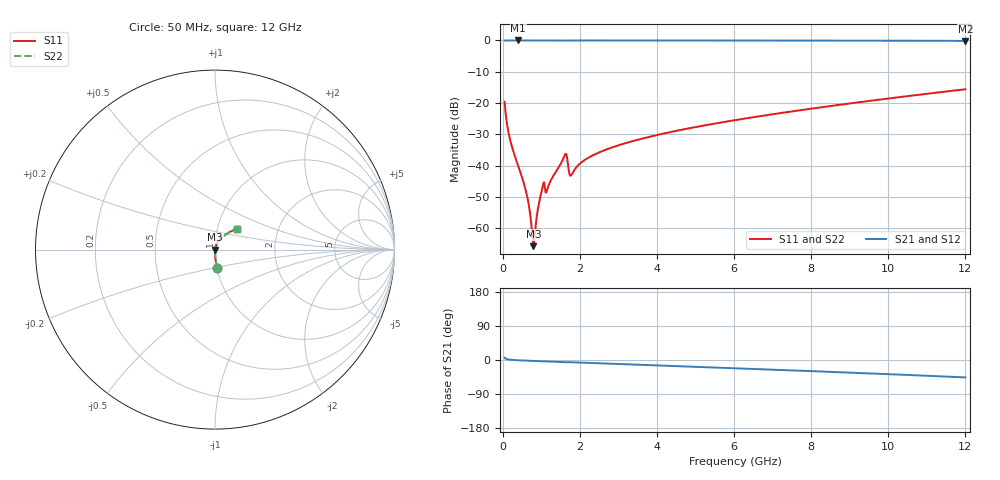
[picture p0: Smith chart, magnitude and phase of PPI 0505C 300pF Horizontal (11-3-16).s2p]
# MHz S MA R 50
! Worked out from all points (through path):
!   1601 points, 50 MHz to 12 GHz, reference 50 ohm
!   highest |S21| = 0.00 dB at 401 MHz (marker M1); lowest = -0.1 dB at 12 GHz (marker M2)
!   group delay of S21, straight-line fit = 10.7 ps
!   lowest |S11| = -65.7 dB at 796.9 MHz (marker M3), VSWR 1.00, Z = 50.1 - j0.00941 ohm
!   |S11| at or under -10 dB: start of sweep to end of sweep
!   |S22| runs from -65.7 to -15.6 dB; largest |S21 - S12| = 0
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50  0.105 -84.0  0.9943 5.9  0.9943 5.9  0.105 -84.0
191.9062  0.02606 -88.5  0.9993 0.9  0.9993 0.9  0.02606 -88.5
401.0312  0.01001 -88.5  0.9995 -0.7  0.9995 -0.7  0.01001 -88.5
625.0938  0.003442 -84.1  0.9995 -1.8  0.9995 -1.8  0.003442 -84.1
684.8438  0.002212 -79.6  0.9995 -2.0  0.9995 -2.0  0.002212 -79.6
759.5312  0.000893 -58.3  0.9995 -2.3  0.9995 -2.3  0.000893 -58.3
796.875  0.0005189 -10.4  0.9994 -2.5  0.9994 -2.5  0.0005189 -10.4
834.2188  0.0007852 44.8  0.9994 -2.7  0.9994 -2.7  0.0007852 44.8
931.3125  0.002338 71.9  0.9993 -3.1  0.9993 -3.1  0.002338 71.9
1035.875  0.004617 70.9  0.9987 -3.5  0.9987 -3.5  0.004617 70.9
1162.844  0.004308 72.4  0.9989 -3.9  0.9989 -3.9  0.004308 72.4
1603.5  0.01447 64.4  0.9949 -5.8  0.9949 -5.8  0.01447 64.4
1648.312  0.01526 45.8  0.9903 -5.9  0.9903 -5.9  0.01526 45.8
1737.938  0.00715 42.7  0.9951 -5.8  0.9951 -5.8  0.00715 42.7
1775.281  0.00704 58.0  0.9968 -5.9  0.9968 -5.9  0.00704 58.0
2044.156  0.01132 77.5  0.9987 -7.1  0.9987 -7.1  0.01132 77.5
2768.625  0.01889 77.5  0.9987 -9.7  0.9987 -9.7  0.01889 77.5
4038.312  0.03123 73.8  0.9983 -14.4  0.9983 -14.4  0.03123 73.8
6025  0.05336 67.0  0.997 -21.8  0.997 -21.8  0.05336 67.0
8019.156  0.08167 59.6  0.9948 -29.4  0.9948 -29.4  0.08167 59.6
10013.31  0.1185 51.8  0.9907 -37.4  0.9907 -37.4  0.1185 51.8
12000  0.1661 43.4  0.9835 -45.9  0.9835 -45.9  0.1661 43.4
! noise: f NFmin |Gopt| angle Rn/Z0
50  0.0003176  0.8364  0.2538  0.0004103
1372  0.003536  0.6402  4.259  0.001853
2701  0.005111  0.5406  8.254  0.001964
4031  0.00665  0.4918  12.11  0.002225
5360  0.008191  0.4643  15.87  0.002535
6682  0.009702  0.4466  19.48  0.002848
8012  0.01123  0.4355  22.97  0.003176
9341  0.01278  0.4296  26.33  0.003527
1.067e+04  0.01439  0.4282  29.56  0.003912
1.2e+04  0.01609  0.4306  32.66  0.004344
